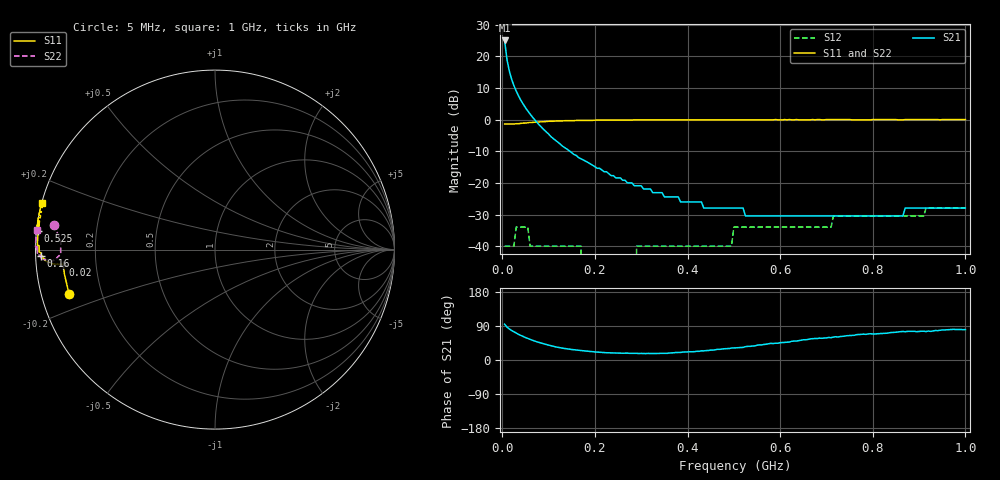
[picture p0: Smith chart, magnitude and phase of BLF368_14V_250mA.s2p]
! Filename:  BLF368_14V_250mA.s2p
! Philips part #: BLF368  !date: 21-05-2003
!14V @250 mA
!D:\Vee measurements\measurement data\VDMOST\BLF368\14V_250mA_#1
# HZ S MA R 50
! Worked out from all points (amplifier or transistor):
!   200 points, 5 MHz to 1 GHz, reference 50 ohm
!   highest |S21| = 25.0 dB at 5 MHz (marker M1)
!   |S21| within 3 dB of that: start of sweep to 7.526 MHz
!   S11 on the Smith chart (normalised r, x): 5 MHz: 0.08, -0.15; 20 MHz: 0.08, -0.05; 160 MHz: 0.02, -0.02; 525 MHz: 0.01, +0.05; 1 GHz: -0.00, +0.13
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5000000  0.85 -163.1  17.77 94.6  0.01 3.5  0.91 171.2
1e7  0.85 -170.8  8.97 87.1  0.01 21.7  0.87 175.5
1.5e7  0.85 -173.2  5.93 82.0  0.01 22.0  0.86 177.3
2e7  0.85 -174.1  4.37 77.9  0.01 18.1  0.86 178.6
2.5e7  0.85 -174.4  3.45 74.5  0.01 13.1  0.86 179.6
3e7  0.86 -174.6  2.83 70.9  0.02 7.8  0.86 -179.8
3.5e7  0.86 -174.6  2.37 67.7  0.02 3.3  0.86 -179.1
5.5e7  0.89 -174.7  1.37 56.8  0.02 -11.0  0.88 -176.9
6e7  0.9 -174.8  1.22 54.3  0.01 -13.8  0.89 -176.6
1e8  0.94 -175.9  0.59 39.2  0.01 -27.9  0.93 -176.1
1.6e8  0.97 -178.0  0.27 26.4  0.01 -26.5  0.96 -176.8
1.7e8  0.97 -178.3  0.24 24.9  0.01 -23.0  0.97 -176.9
1.75e8  0.97 -178.5  0.23 24.4  0 -20.8  0.97 -177.0
2.85e8  0.99 178.6  0.09 17.4  0 68.2  0.99 -179.0
2.9e8  0.99 178.5  0.09 17.5  0.01 69.8  0.99 -179.1
3.4e8  0.99 177.5  0.07 17.5  0.01 76.5  0.99 -179.7
4.95e8  0.99 174.4  0.04 31.6  0.01 88.4  1 178.5
5.05e8  0.99 174.2  0.04 32.1  0.02 88.3  1 178.4
5.25e8  0.99 173.9  0.03 35.3  0.02 88.7  1 178.3
6.7e8  1 171.3  0.03 56.2  0.02 90.4  1 176.8
8.35e8  1 168.2  0.03 71.5  0.03 92.6  1 175.3
1e9  1 165.1  0.04 80.3  0.04 91.5  1 173.6
